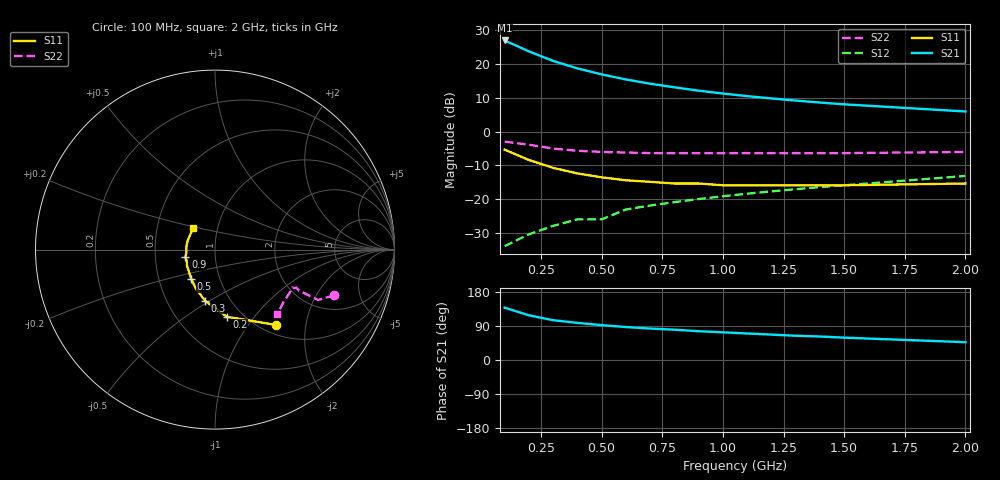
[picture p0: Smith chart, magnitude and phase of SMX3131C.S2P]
! HSMX-3131 Common Emitter
! Vce=10V Ic=15ma
# ghz s ma r 50
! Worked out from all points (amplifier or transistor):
!   16 points, 100 MHz to 2 GHz, reference 50 ohm
!   highest |S21| = 27.0 dB at 100 MHz (marker M1)
!   |S21| within 3 dB of that: start of sweep to 192.8 MHz
!   unconditionally stable (mu >= 1): 441.7 MHz to 1.824 GHz
!   at 300 MHz: K = 0.85, MSG = 24.5 dB, |S12| = -28.0 dB
!   at 900 MHz: K = 1.05, MAG = 14.8 dB, |S12| = -20.0 dB
!   at 2 GHz: K = 0.97, MSG = 9.6 dB, |S12| = -13.2 dB
!   S11 on the Smith chart (normalised r, x): 100 MHz: 1.16, -1.37; 200 MHz: 0.85, -0.74; 300 MHz: 0.77, -0.48; 500 MHz: 0.73, -0.25; 900 MHz: 0.71, -0.06; 2 GHz: 0.76, +0.19
0.1  0.54 -51.0  22.5 138.0  0.02 70.0  0.71 -21.0
0.2  0.38 -80.0  15.51 118.0  0.03 67.0  0.64 -26.0
0.3  0.29 -101.0  11.18 105.0  0.04 68.0  0.56 -26.0
0.4  0.24 -117.0  8.67 98.0  0.05 70.0  0.52 -26.0
0.5  0.21 -129.0  7.06 92.0  0.05 71.0  0.5 -25.0
0.6  0.19 -140.0  5.94 87.0  0.07 72.0  0.49 -26.0
0.7  0.18 -150.0  5.14 83.0  0.08 72.0  0.48 -26.0
0.8  0.17 -158.0  4.54 80.0  0.09 73.0  0.48 -27.0
0.9  0.17 -166.0  4.05 76.0  0.1 73.0  0.48 -29.0
1  0.16 -173.0  3.67 73.0  0.11 73.0  0.48 -30.0
1.1  0.16 -179.0  3.36 70.0  0.12 73.0  0.48 -31.0
1.2  0.16 175.0  3.11 67.0  0.13 72.0  0.48 -33.0
1.3  0.16 170.0  2.89 64.0  0.14 72.0  0.48 -34.0
1.4  0.16 164.0  2.7 62.0  0.15 71.0  0.48 -36.0
1.5  0.16 159.0  2.54 59.0  0.16 71.0  0.48 -37.0
2  0.17 136.0  1.99 47.0  0.22 68.0  0.5 -46.0
